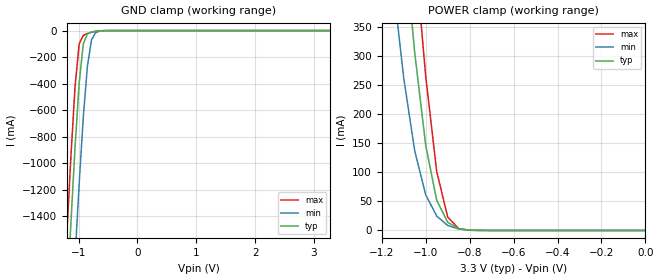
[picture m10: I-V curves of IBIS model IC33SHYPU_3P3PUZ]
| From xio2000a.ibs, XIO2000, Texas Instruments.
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|   Model IC33SHYPU_3P3PUZ
[Model]   IC33SHYPU_3P3PUZ
Model_type   Input
Polarity   Non-Inverting
Vinl =   0.9900V
Vinh =   2.3100V
C_comp   2.0800pF   2.0800pF   2.0800pF
[Temperature Range]   25.0000   0.1250k   -40.0000
[Voltage Range]   3.3000V   3.0000V   3.6000V
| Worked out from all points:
|   GND clamp passes 1 mA (typ) near -0.59 V on its own axis
|   POWER clamp passes 1 mA (typ) near -0.81 V on its own axis
[GND_clamp]
| voltage   I(typ)   I(min)   I(max)
-3.3V     -22.44A    -23.23A    -22.01A
-1.2V     -2.062A    -2.938A    -1.55A
-1.13V    -1.453A    -2.319A    -952mA
-1.06V    -884.2mA   -1.722A    -426.9mA
-990mV    -399.1mA   -1.159A    -102.2mA
-920mV    -101.9mA   -657.3mA   -35.64mA
-850mV    -24.64mA   -270.7mA   -22.38mA
-780mV    -11.46mA   -69.99mA   -12.94mA
-710mV    -5.643mA   -15.28mA   -5.841mA
-640mV    -2.142mA   -4.297mA   -1.755mA
3.28V     182.6pA    7.2nA      156.8pA
[POWER_clamp]
| voltage   I(typ)   I(min)   I(max)
-3.3V     12.64A     11.74A     13.39A
-1.15V    732.9mA    428mA      979.8mA
-1.1V     506.3mA    260.8mA    722.9mA
-1.05V    304.4mA    136.2mA    480.2mA
-1V       145.7mA    61.22mA    263.9mA
-950mV    51.67mA    24.6mA     101mA
-900mV    14.1mA     8.528mA    22.97mA
-850mV    2.852mA    2.481mA    3.15mA
-800mV    471.8uA    685uA      302.8uA
-750mV    76.23uA    214.3uA    28.26uA
0V        184.8pA    2.737nA    176.4pA
